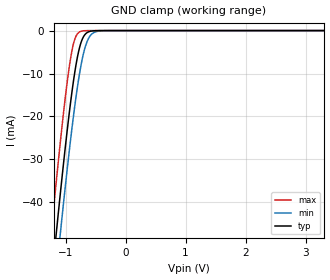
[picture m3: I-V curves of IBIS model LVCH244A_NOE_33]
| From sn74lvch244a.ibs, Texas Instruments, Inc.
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[Model]   LVCH244A_NOE_33
Model_type  Input
Vinl=0.8
Vinh=2.0
| variable   typ   min   max
C_comp   3.37pF   3.00pF   3.86pF
[Temperature Range]   40   100   -40
| Ambient temperature   25   85   -40
[Voltage range]   3.3   3   3.6
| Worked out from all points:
|   GND clamp passes 1 mA (typ) near -0.68 V on its own axis
[GND Clamp]
| LVCH244A_NOE_33
|   Voltage   I(typ)   I(min)   I(max)
-5.5V     -731.8mA   -738.6mA   -723.7mA
-1.25V    -60.73mA   -70.05mA   -48.77mA
-1.22V    -56.44mA   -65.77mA   -44.44mA
-1.145V   -45.9mA    -55.24mA   -33.86mA
-1.095V   -39.06mA   -48.38mA   -27.07mA
-1.075V   -36.38mA   -45.67mA   -24.43mA
-950mV    -20.6mA    -29.51mA   -9.641mA
-855mV    -10.53mA   -18.51mA   -2.421mA
-775mV    -4.434mA   -10.71mA   -383.6uA
-705mV    -1.535mA   -5.568mA   -59.89uA
-555mV    -87.15uA   -716.5uA   -1.006uA
3.3V      1.117nA    59.62nA    9.38pA
